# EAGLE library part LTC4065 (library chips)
LION/LIPO Battery Charging IC Low current
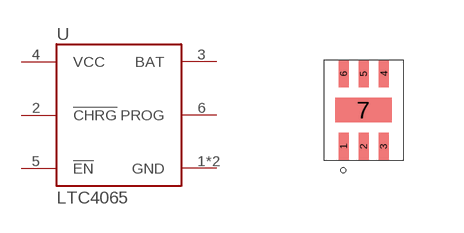
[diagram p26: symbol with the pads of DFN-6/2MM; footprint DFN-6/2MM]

Designator prefix -

## LTC4065 (DIGIKEY: LTC4065LEDC#TRMPBF)  [DFN-6/2MM]
1  GND
2  !CHRG
3  BAT
4  VCC
5  !EN
6  PROG
7  GND

## Footprint DFN-6/2MM (pad centres in mm)
smd 0.25 x 0.675: 1 -0.5,-0.91; 2 0,-0.91; 3 0.5,-0.91; 4 0.51,0.91; 5 0,0.91; 6 -0.5,0.91
smd 1.42 x 0.61: 7 0,0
